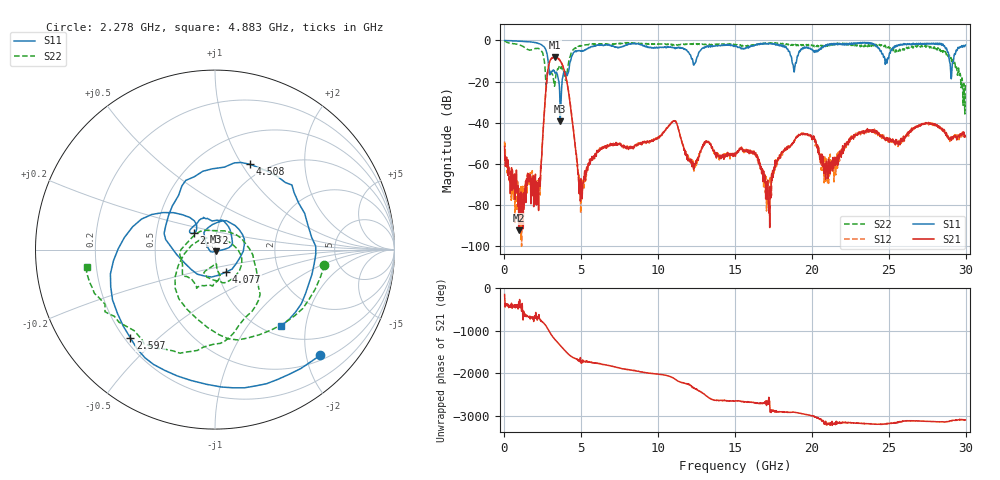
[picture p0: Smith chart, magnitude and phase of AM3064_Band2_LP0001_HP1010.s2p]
# Hz S DB R 50.0
!freq dBS11 angS11 dBS21 angS21 dBS12 angS12 dBS22 angS22
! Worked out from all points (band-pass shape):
!   1600 points, 10 MHz to 29.98 GHz, reference 50 ohm
!   highest |S21| = -8.03 dB at 3.271 GHz (marker M1); lowest = -92.3 dB at 928.4 MHz (marker M2)
!   |S21| within 3 dB of the highest: 2.912 GHz to 3.715 GHz (802.4 MHz wide, 24.2 % of centre)
!   lowest |S11| = -39.4 dB at 3.628 GHz (marker M3), VSWR 1.02, Z = 50.6 - j0.882 ohm
!   |S11| at or under -10 dB: 2.837 GHz to 4.297 GHz (1.46 GHz wide, 40.9 % of centre); 18.7 GHz to 19 GHz (297 MHz wide, 1.58 % of centre); 28.94 GHz to 29.2 GHz (257.1 MHz wide, 0.884 % of centre)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
!   |S22| runs from -35.7 to -0.2 dB; largest |S21 - S12| = 0.01
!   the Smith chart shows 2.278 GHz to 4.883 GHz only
!   S11 on the Smith chart (normalised r, x): 2.278 GHz: 0.60, -2.27; 2.597 GHz: 0.22, -0.41; 2.972 GHz: 0.78, +0.15; 4.077 GHz: 1.09, -0.28; 4.508 GHz: 0.84, +1.09; 4.883 GHz: 1.18, -1.47
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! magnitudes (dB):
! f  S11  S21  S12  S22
! 10 MHz  0.0  -51.5  -49.2  -0.2
! 928.4 MHz  -0.4  -92.3  -81.3  -2.1
! 2.278 GHz  -1.6  -68.4  -68.3  -4.2
! 2.597 GHz  -3.3  -34.4  -34.3  -10.2
! 2.972 GHz  -16.5  -9.7  -9.7  -15.0
! 3.271 GHz  -15.4  -8.0  -8.0  -21.7
! 3.628 GHz  -39.4  -9.8  -9.7  -13.3
! 4.077 GHz  -17.1  -20.9  -20.9  -15.3
! 4.508 GHz  -5.8  -44.9  -44.9  -4.3
! 4.883 GHz  -5.0  -68.7  -68.7  -2.9
! 5.015 GHz  -5.4  -72.5  -69.7  -2.6
! 6.289 GHz  -2.1  -52.6  -52.7  -1.7
! 10 GHz  -3.5  -47.2  -46.9  -1.7
! 15 GHz  -2.6  -56.2  -55.0  -1.9
! 16.32 GHz  -2.2  -55.0  -55.6  -1.9
! 17.2 GHz  -1.5  -83.8  -76.3  -1.6
! 18.12 GHz  -3.2  -54.4  -55.1  -1.5
! 19.99 GHz  -4.3  -46.7  -47.0  -2.2
! 21.02 GHz  -1.8  -61.5  -69.8  -2.5
! 25 GHz  -8.3  -48.7  -47.7  -3.1
! 28.56 GHz  -2.5  -43.7  -43.2  -5.0
! 29.98 GHz  -2.3  -46.8  -46.4  -21.7
